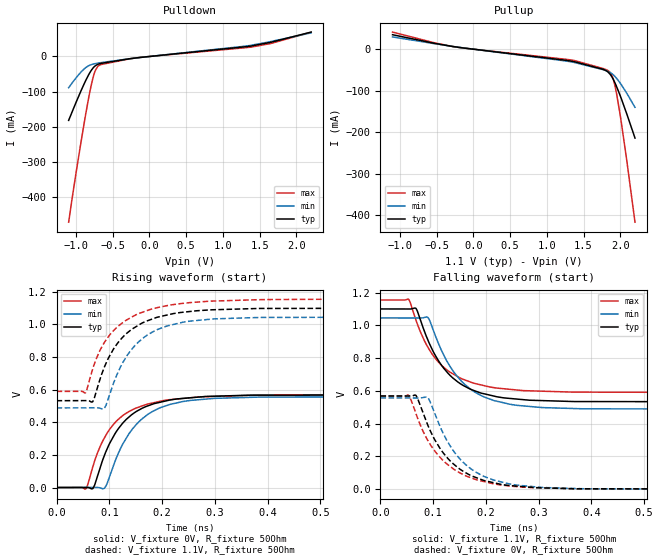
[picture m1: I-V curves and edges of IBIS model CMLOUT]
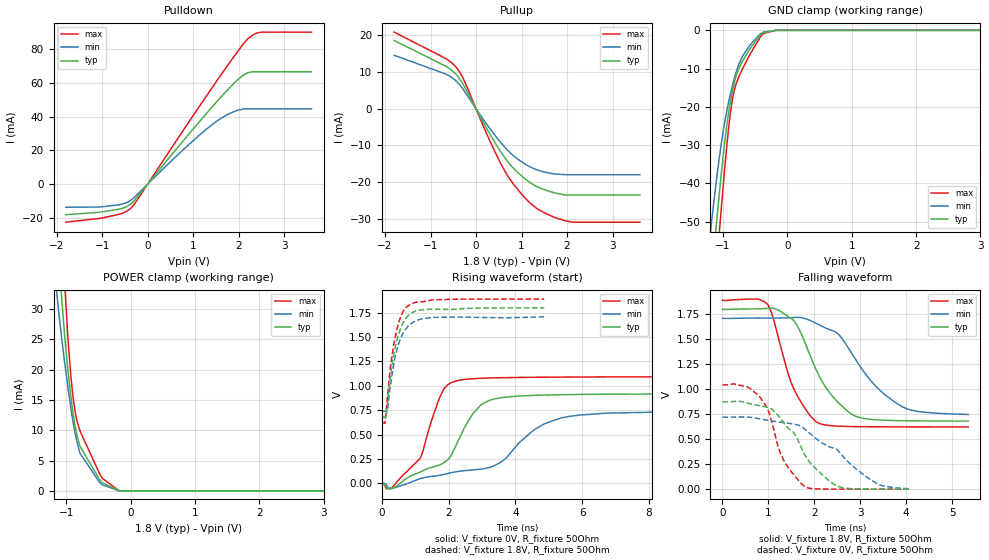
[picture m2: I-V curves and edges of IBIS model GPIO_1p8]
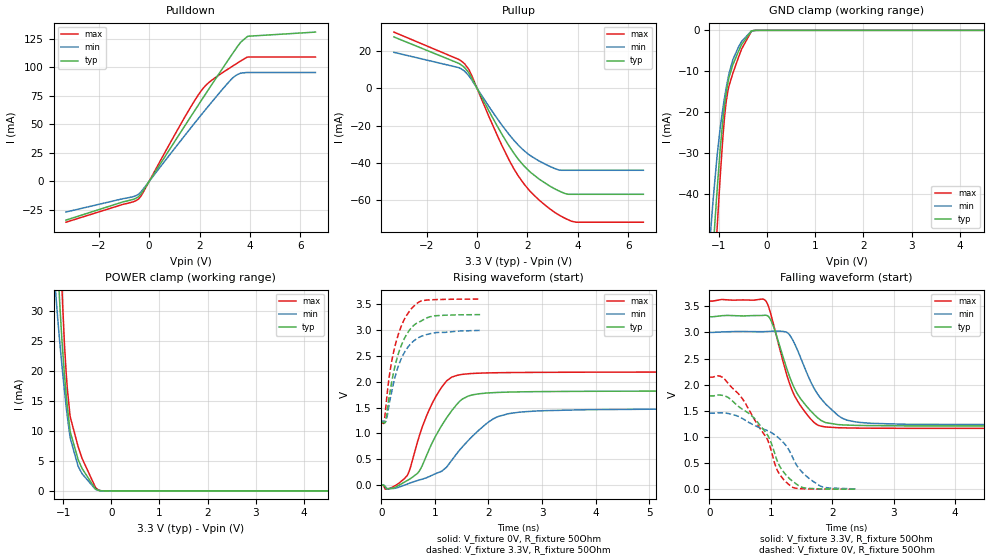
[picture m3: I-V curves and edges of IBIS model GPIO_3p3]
| Texas Instruments Incorporated
| DS90UB9702-Q1 FPD-Link III/IV QuadDeserializer with MIPICSI-2 DPHY out. ports
| Marketing part#   Digital Voltage Range   Package-type   #pins
| DS90UB9702-Q1   1.1V - 3.6V   VQFNP   88
[IBIS Ver]   4.1
[File name]   ds90ub9702-q1.ibs
[File Rev]   1.0
[Date]   05/27/2021
[Source]
| Texas Instruments Incorporated.
| FPD-Link Design and Systems Engineering
| 2900 Semiconductor Driver
| Santa Clara, CA
[Notes]   Revision History:
| Rev 1.0: 05/27/2021
| - Initial version of the model
| - Model generated from simulations in CADENCE
| - Warnings regarding combined Non-monotonicity of various models
|   have been reviewed and considered minor and can be ignored.
| - FPD3_RX, FPD4_RX used in single ended mode
[Disclaimer]
| This model is designed as an aid for customers of Texas Instruments.
| TI and its licensors and suppliers make no warranties, either expressed
| or implied, with respect to this  model, including the warranties of
| merchantability or fitness for a particular purpose. The model is
| provided solely on an "as is" basis. The entire risk as to its quality
| and performance is with the customer.
[Copyright]
(C) Copyright 2021 Texas Instruments Incorporated.All rights reserved.
|   ds90ub9702-q1
[Component]   ds90ub9702-q1
[Manufacturer]   TI
[Package]   |VQFNP 88
|   typ   min   max
R_pkg   0.117   0.089   0.157
L_pkg   2.39nH   1.95nH   3.04nH
C_pkg   0.493pF   0.405pF   0.603pF
[Pin] signal_name  model_name   R_pin  L_pin  C_pin
  1   CML2P   CMLOUT   NA   NA   NA
  2   CML2N   CMLOUT   NA   NA   NA
  3   CML3P   CMLOUT   NA   NA   NA
  4   CML3N   CMLOUT   NA   NA   NA
  5   VDD11_L   power   NA   NA   NA
  6   GPIO0   GPIO   NA   NA   NA
  7   GPIO1   GPIO   NA   NA   NA
  8   GPIO2   GPIO   NA   NA   NA
  9   INTB/GPIO3   GPIO2   NA   NA   NA
 10   LOCK/GPIO4   GPIO   NA   NA   NA
 11   GPIO5   GPIO   NA   NA   NA
 12   GPIO6   GPIO   NA   NA   NA
 13   GPIO7   GPIO   NA   NA   NA
 14   RES   nc   NA   NA   NA
 15   REFCLK   REFCLK   NA   NA   NA
 16  VDDIO   power   NA   NA   NA
 17  CSI2_CLK0N   DPHYTX   NA   NA   NA
 18  CSI2_CLK0P   DPHYTX   NA   NA   NA
 19  CSI2_D0N   DPHYTX   NA   NA   NA
 20  CSI2_D0P   DPHYTX   NA   NA   NA
 21  CSI2_D1N   DPHYTX   NA   NA   NA
 22  CSI2_D1P   DPHYTX   NA   NA   NA
 23  CSI2_CLK1N   DPHYTX   NA   NA   NA
 24  CSI2_CLK1P   DPHYTX   NA   NA   NA
 25  CSI2_D2N   DPHYTX   NA   NA   NA
 26  CSI2_D2P   DPHYTX   NA   NA   NA
 27  CSI2_D3N   DPHYTX   NA   NA   NA
 28  CSI2_D3P   DPHYTX   NA   NA   NA
 29  VDD11_CSI   power   NA   NA   NA
 30  VDD11_CSI   power   NA   NA   NA
 31  CSI0_CLK0N   DPHYTX   NA   NA   NA
 32  CSI0_CLK0P   DPHYTX   NA   NA   NA
 33  CSI0_D0N   DPHYTX   NA   NA   NA
 34  CSI0_D0P   DPHYTX   NA   NA   NA
 35  CSI0_D1N   DPHYTX   NA   NA   NA
 36  CSI0_D1P   DPHYTX   NA   NA   NA
 37  CSI0_CLK1N   DPHYTX   NA   NA   NA
 38  CSI0_CLK1P   DPHYTX   NA   NA   NA
 39  CSI0_D2N   DPHYTX   NA   NA   NA
 40  CSI0_D2P   DPHYTX   NA   NA   NA
 41  CSI0_D3N   DPHYTX   NA   NA   NA
 42  CSI0_D3P   DPHYTX   NA   NA   NA
 43  VDD11_CSI   power   NA   NA   NA
 44  VDD18_P   power   NA   NA   NA
 45  VDD11_P   power   NA   NA   NA
 46  VDD11_CSI   power   NA   NA   NA
 47  CSI1_CLK0N   DPHYTX   NA   NA   NA
 48  CSI1_CLK0P   DPHYTX   NA   NA   NA
 49  CSI1_D0N   DPHYTX   NA   NA   NA
 50  CSI1_D0P   DPHYTX   NA   NA   NA
 51  CSI1_D1N   DPHYTX   NA   NA   NA
 52  CSI1_D1P   DPHYTX   NA   NA   NA
 53  CSI1_CLK1N   DPHYTX   NA   NA   NA
 54  CSI1_CLK1P   DPHYTX   NA   NA   NA
 55  CSI1_D2N   DPHYTX   NA   NA   NA
 56  CSI1_D2P   DPHYTX   NA   NA   NA
 57  CSI1_D3N   DPHYTX   NA   NA   NA
 58  CSI1_D3P   DPHYTX   NA   NA   NA
 59  VDD11_CSI   power   NA   NA   NA
 60  TESTEN   nc   NA   NA   NA
 61  PDB   PDB_18   NA   NA   NA
 62  VDD11_L   power   NA   NA   NA
 63  CML0N   CMLOUT   NA   NA   NA
 64  CML0P   CMLOUT   NA   NA   NA
 65  CML1N   CMLOUT   NA   NA   NA
 66  CML1P   CMLOUT   NA   NA   NA
 67  I2C_SDA   I2C   NA   NA   NA
 68  I2C_SCL   I2C   NA   NA   NA
 69  VDD18_FPD0   power   NA   NA   NA
 70  RIN0+   RIN   NA   NA   NA
 71  RIN0-   RIN   NA   NA   NA
 72  VDD11_FPD   power   NA   NA   NA
 73  RIN1+   RIN   NA   NA   NA
 74  RIN1-   RIN   NA   NA   NA
 75  VDD18_FPD1   power   NA   NA   NA
 76  IDX   nc   NA   NA   NA
 77  LPF   nc   NA   NA   NA
 78  MODE   nc   NA   NA   NA
 79  VDD11_CSI   power   NA   NA   NA
 80  VDD18_FPD2   power   NA   NA   NA
 81  RIN2+   RIN   NA   NA   NA
 82  RIN2-   RIN   NA   NA   NA
 83  VDD11_FPD   power   NA   NA   NA
 84  RIN3+   RIN   NA   NA   NA
 85  RIN3-   RIN   NA   NA   NA
 86  VDD18_FPD3   power   NA   NA   NA
 87  I2C_SCL1/GPIO9  I2C1   NA   NA   NA
 88  I2C_SDA1/GPIO10 I2C1   NA   NA   NA
| RIN model the diff cell line in IBIS needs to be commented
| out to use this model
[Diff pin]  inv_pin  vdiff  tdelay_typ  tdelay_min  tdelay_max
  1   2   0.9   0.0s   0.0s   0.0s
  3   4   0.9   0.0s   0.0s   0.0s
  18  17   0.4   0.0s   0.0s   0.0s
  20  19   0.4   0.0s   0.0s   0.0s
  22  21   0.4   0.0s   0.0s   0.0s
  24  23   0.4   0.0s   0.0s   0.0s
  26  25   0.4   0.0s   0.0s   0.0s
  28  27   0.4   0.0s   0.0s   0.0s
  32  31   0.4   0.0s   0.0s   0.0s
  34  33   0.4   0.0s   0.0s   0.0s
  36  35   0.4   0.0s   0.0s   0.0s
  38  37   0.4   0.0s   0.0s   0.0s
  40  39   0.4   0.0s   0.0s   0.0s
  42  41   0.4   0.0s   0.0s   0.0s
  48  47   0.4   0.0s   0.0s   0.0s
  50  49   0.4   0.0s   0.0s   0.0s
  52  51   0.4   0.0s   0.0s   0.0s
  54  53   0.4   0.0s   0.0s   0.0s
  56  55   0.4   0.0s   0.0s   0.0s
  58  57   0.4   0.0s   0.0s   0.0s
  64  63   0.9   0.0s   0.0s   0.0s
  66  65   0.9   0.0s   0.0s   0.0s
 | 70  71   0.4   0.0s   0.0s   0.0s
 | 73  74   0.4   0.0s   0.0s   0.0s
 | 81  82   0.4   0.0s   0.0s   0.0s
 | 84  85   0.4   0.0s   0.0s   0.0s
|   Model Selectors
[Model Selector] GPIO
GPIO_1p8   1.8V  digital GPIO
GPIO_3p3   3.3V  digital GPIO
[Model Selector] GPIO2
INTB_SHAREIO_18   1.8V digital IO Open Drain Cell
INTB_SHAREIO_33   3.3V digital IO Open Drain Cell
IO_SHAREINTB_18   1.8V digital GPIO for combination with Open Drain Cell
IO_SHAREINTB_33   3.3V digital GPIO for combination with Open Drain Cell
[Model Selector] REFCLK
REFCLK_18   REFCLK 1.8v
REFCLK_33   REFCLK 3.3v
[Model Selector] I2C
I2C_FAST_33   I2C FAST 3.3v
I2C_FAST_18   I2C FAST 1.8v
I2C_FASTPLUS_33   I2C FASTPLUS 3.3v
I2C_FASTPLUS_18   I2C FASTPLUS 1.8v
[Model Selector] I2C1
I2C_FAST_33   I2C FAST 3.3v
I2C_FAST_18   I2C FAST 1.8v
I2C_FASTPLUS_33   I2C FASTPLUS 3.3v
I2C_FASTPLUS_18   I2C FASTPLUS 1.8v
GPIO2_1p8   1.8V digital GPIO for combination with Open Drain Cell
GPIO2_3p3   1.8V digital GPIO for combination with Open Drain Cell
[Model Selector] DPHYTX
DPHY_HS   DPHY Tx HS
DPHY_LP   DPHY Tx LP
[Model Selector] RIN
FPD3_RX   FPD-Link 3 Receiver-Transmitter
FPD4_RX   FPD-Link 4 Receiver-Transmitter
| Models and submodels in the file (20): CMLOUT (Output), GPIO_1p8 (I/O), GPIO_3p3 (I/O), GPIO2_1p8 (I/O), GPIO2_3p3 (I/O), REFCLK_18 (Input), REFCLK_33 (Input), I2C_FAST_18 (I/O_open_drain), I2C_FAST_33 (I/O_open_drain), I2C_FASTPLUS_18 (I/O_open_drain), I2C_FASTPLUS_33 (I/O_open_drain), PDB_18 (Input), DPHY_HS (Output), DPHY_LP (Output), INTB_SHAREIO_18 (I/O_open_drain), INTB_SHAREIO_33 (I/O_open_drain), IO_SHAREINTB_18 (I/O), IO_SHAREINTB_33 (I/O), FPD3_RX (I/O), FPD4_RX (I/O)
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|   CMLOUT Model
[Model]   CMLOUT
Model_type   Output
Polarity   Non-Inverting
Vmeas = 0.55
Vref = 0.55
Cref = 0pF
Rref = 50
|   typ   min   max
C_comp   1.329pF   1.392pF   1.158pF
[Voltage Range]   1.1   1.045   1.155
[Temperature Range]   27   105   -40
[Pullup Reference]   1.1   1.045   1.155
[Pulldown Reference]   -0   -0   0
[Power Clamp Reference]   1.1   1.045   1.155
[GND Clamp Reference]   0   0   0
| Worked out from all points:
|   slope of the pulldown table from 0 to 0.165 V, typ, clamps not added: 46.5 ohm
|   slope of the pullup table from 0 to 0.165 V, typ, clamps not added: 46.5 ohm
|   falling waveform, V_fixture 1.1V, R_fixture 50Ohm: 20-80 % time 69.8ps typ, 71.3ps min, 72.1ps max; typ from 1.1 V to 0.532 V
|   rising waveform, V_fixture 0V, R_fixture 50Ohm: 20-80 % time 64.2ps typ, 66.4ps min, 64.3ps max; typ from 0.001 V to 0.569 V
|   rising waveform, V_fixture 1.1V, R_fixture 50Ohm: 20-80 % time 70.5ps typ, 67.9ps min, 74.8ps max; typ from 0.532 V to 1.1 V
|   falling waveform, V_fixture 0V, R_fixture 50Ohm: 20-80 % time 72.5ps typ, 72.3ps min, 75.1ps max; typ from 0.569 V to 0.001 V
[Pulldown]
|   Voltage   I(typ)   I(min)   I(max)
-1.1V     -182.3mA   -89mA      -472.7mA
-1.05V    -156.9mA   -74.89mA   -401.7mA
-931.7mV  -97.86mA   -44.34mA   -243.8mA
-829.4mV  -52.8mA    -26.56mA   -120.1mA
-793.1mV  -39.97mA   -23.28mA   -82.45mA
-756.8mV  -30.23mA   -21.16mA   -52.03mA
-737mV    -26.5mA    -20.27mA   -40.1mA
-694.1mV  -21.7mA    -18.66mA   -26.62mA
-136.4mV  -3.021mA   -3.195mA   -2.891mA
1.382V    29.73mA    31.87mA    26.64mA
1.662V    41.07mA    43.15mA    37.62mA
2.2V      69.57mA    67.39mA    69.39mA
[Pullup]
|   Voltage   I(typ)   I(min)   I(max)
-1.1V     34.88mA    29.53mA    41.23mA
-235.4mV  5.289mA    5.509mA    5.07mA
1.335V    -29.01mA   -30.79mA   -26.25mA
1.764V    -48.67mA   -49.31mA   -46.6mA
1.83V     -54.84mA   -53.46mA   -51.41mA
1.86V     -60.26mA   -56.13mA   -55.69mA
1.893V    -69.21mA   -60.2mA    -66.46mA
1.923V    -79.58mA   -65.05mA   -84.76mA
1.949V    -90.16mA   -70.26mA   -107.3mA
2.012V    -118.5mA   -85.19mA   -174.6mA
2.091V    -157.7mA   -107.2mA   -272.5mA
2.2V      -214.5mA   -140.3mA   -417.4mA
[Ramp]
R_load = 50
|   typ   min   max
dV/dt_r   0.341018/6.43645e-11   0.333768/6.66287e-11   0.340926/6.43299e-11
dV/dt_f   0.340493/6.98585e-11   0.334059/7.13859e-11   0.339127/7.12696e-11
[Falling Waveform]
V_fixture = 1.1V
V_fixture_min = 1.045V
V_fixture_max = 1.155V
R_fixture = 50Ohm
C_fixture = 0F
|   Time   V(typ)   V(min)   V(max)
0s        1.1V       1.045V     1.154V
53.68ps   1.099V     1.045V     1.158V
67.79ps   1.102V     1.045V     1.029V
89.79ps   912.7mV    1.049V     868.1mV
113.7ps   766.3mV    862.1mV    763.2mV
140.1ps   671.9mV    711.6mV    699.3mV
171ps     610.4mV    610.6mV    654mV
207ps     574.6mV    550.8mV    624.2mV
384.8ps   534.9mV    490.7mV    592.2mV
1ns       532.3mV    488.1mV    589.2mV
[Rising Waveform]
V_fixture = 0V
V_fixture_min = 0V
V_fixture_max = 0V
R_fixture = 50Ohm
C_fixture = 0F
|   Time   V(typ)   V(min)   V(max)
0s        540.9uV    677.7uV    610.6uV
55.55ps   1.062mV    1.133mV    -7.529mV
69.19ps   -4.06mV    1.245mV    131.9mV
90.63ps   196.2mV    -4.053mV   304mV
113.7ps   345.1mV    184.3mV    407.7mV
140.1ps   440mV      342.7mV    470.4mV
171ps     498.1mV    443.7mV    510.1mV
200.6ps   525.9mV    493.7mV    531.7mV
384.8ps   566.1mV    554.4mV    565.9mV
1ns       568.9mV    557mV      568.8mV
[Rising Waveform]
V_fixture = 1.1V
V_fixture_min = 1.045V
V_fixture_max = 1.155V
R_fixture = 50Ohm
C_fixture = 0F
|   Time   V(typ)   V(min)   V(max)
0s        532.2mV    488.1mV    589.2mV
54.91ps   532.7mV    488.5mV    580.6mV
68.52ps   525.9mV    488.6mV    726mV
89.79ps   730.4mV    482.7mV    883.6mV
120ps     901.1mV    731mV      996.6mV
140.1ps   963.1mV    837.3mV    1.039V
175.2ps   1.025V     940.7mV    1.088V
221.3ps   1.065V     998.7mV    1.121V
384.8ps   1.097V     1.042V     1.151V
1ns       1.1V       1.045V     1.154V
[Falling Waveform]
|Gnd
V_fixture = 0V
V_fixture_min = 0V
V_fixture_max = 0V
R_fixture = 50Ohm
C_fixture = 0F
|   Time   V(typ)   V(min)   V(max)
0s        568.9mV    557mV      568.8mV
53.37ps   568.6mV    556.8mV    573.8mV
67.98ps   569.9mV    556.7mV    457mV
89.29ps   396mV      561mV      301.3mV
113.7ps   246mV      378.3mV    193mV
143.7ps   140.6mV    211.8mV    113.4mV
175.2ps   78.68mV    116.6mV    65.93mV
213.7ps   40.69mV    57.28mV    33.78mV
384.8ps   2.882mV    3.195mV    2.937mV
1ns       541uV      676.8uV    609.5uV
|   GPIO_1p8 Model
[Model]   GPIO_1p8
Model_type   I/O
Polarity   Non-Inverting
Enable   Active-Low
Vinl = 0.63
Vinh = 1.17
Vmeas = 0.9
Vref = 0
Cref = 2pF
Rref = 80
|   typ   min   max
|   (nom PVT)   (fast PVT)   (slow PVT)
C_comp   3.718e-13   3.701e-13   4.153e-13
| Where nom  PVT is Nominal Process, 1.8V, 27C
|   Fast PVT is Strong Process,  1.89V, -40C
|   Slow PVT is Weak Process,   1.71V, 125C
[Voltage Range]   1.8   1.71   1.89
|Junction Temperature
[Temperature Range]   27   125   -40
[Pullup Reference]   1.8   1.71   1.89
[Pulldown Reference]   0   0   0
[Power Clamp Reference]   1.8   1.71   1.89
[GND Clamp Reference]   0   0   0
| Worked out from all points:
|   slope of the pulldown table from 0 to 0.27 V, typ, clamps not added: 30.2 ohm
|   slope of the pullup table from 0 to 0.27 V, typ, clamps not added: 43.9 ohm
|   GND clamp passes 1 mA (typ) near -0.40 V on its own axis
|   falling waveform, V_fixture 1.8V, R_fixture 50Ohm: 20-80 % time 748ps typ, 967ps min, 555ps max; typ from 1.8 V to 0.682 V
|   rising waveform, V_fixture 0V, R_fixture 50Ohm: 20-80 % time 1.1ns typ, 1.78ns min, 675ps max; typ from 0 V to 0.874 V
|   rising waveform, V_fixture 1.8V, R_fixture 50Ohm: 20-80 % time 358ps typ, 369ps min, 331ps max; typ from 0.681 V to 1.8 V
|   falling waveform, V_fixture 0V, R_fixture 50Ohm: 20-80 % time 824ps typ, 1.21ns min, 503ps max; typ from 0.875 V to 0 V
[Pulldown]
|   Voltage   I(typ)   I(min)   I(max)
-1.8V     -18.1mA    -13.7mA    -22.52mA
-1.118V   -16.75mA   -13.57mA   -20.48mA
-616.7mV  -14.76mA   -12.18mA   -17.81mA
-370.8mV  -11.74mA   -9.537mA   -14.3mA
682.9mV   22.51mA    17.91mA    27.88mA
1.375V    44.46mA    34.38mA    55.51mA
1.806V    57.22mA    41.87mA    72.16mA
2.108V    64.69mA    44.51mA    83.23mA
2.222V    66.11mA    44.62mA    86.57mA
2.351V    66.54mA    44.62mA    88.92mA
2.507V    66.54mA    44.62mA    90.02mA
3.6V      66.54mA    44.62mA    90.04mA
[GND Clamp]
|   Voltage   I(typ)   I(min)   I(max)
-1.8V     -186.8mA   -154.6mA   -219.7mA
-1.184V   -65.39mA   -50.91mA   -80.03mA
-1.142V   -57.47mA   -44.58mA   -70.68mA
-1.093V   -48.73mA   -37.8mA    -60.24mA
-1.032V   -38.28mA   -30.14mA   -47.51mA
-918mV    -21.99mA   -19.11mA   -26.27mA
-867.6mV  -16.94mA   -15.37mA   -19.43mA
-826.6mV  -13.75mA   -12.69mA   -15.72mA
-692.5mV  -7.885mA   -6.615mA   -9.905mA
-371.2mV  -556.1uA   -459.4uA   -815.6uA
-180mV    -2.088uA   -5.52uA    -1.102uA
3.6V      0A         0A         0A
[Pullup]
|   Voltage   I(typ)   I(min)   I(max)
-1.8V     18.57mA    14.55mA    20.87mA
-687.6mV  11.7mA     9.532mA    13.79mA
-427.9mV  9.197mA    7.405mA    11.15mA
-295.6mV  6.918mA    5.493mA    8.587mA
252mV     -5.809mA   -4.572mA   -7.364mA
467.5mV   -10.33mA   -8.117mA   -13.11mA
628.7mV   -13.33mA   -10.48mA   -16.92mA
951.8mV   -17.82mA   -14.11mA   -22.6mA
1.319V    -21.16mA   -16.61mA   -27.08mA
1.761V    -23.08mA   -17.88mA   -29.82mA
2.117V    -23.57mA   -18.03mA   -30.96mA
3.6V      -23.57mA   -18.03mA   -30.98mA
[POWER Clamp]
|   Voltage   I(typ)   I(min)   I(max)
-1.8V     198.5mA    148.8mA    248.5mA
-1.154V   45.96mA    33.07mA    64.85mA
-1.133V   41.99mA    30.87mA    59.48mA
-1.076V   32.34mA    25.46mA    45.52mA
-1.018V   24.38mA    20.39mA    32.58mA
-930.6mV  15.62mA    13.69mA    19.01mA
-889mV    12.28mA    10.92mA    14.86mA
-849.6mV  9.776mA    8.708mA    12.16mA
-783.2mV  7.264mA    6.117mA    9.767mA
-443mV    1.357mA    1.021mA    2.096mA
-180mV    9.68uA     16.22uA    11.61uA
3.6V      0A         0A         0A
[Ramp]
R_load = 50
|   typ   min   max
dV/dt_r   0.524217/1.09833e-09   0.43397/1.76732e-09   0.626665/6.67214e-10
dV/dt_f   0.671532/7.48876e-10   0.581643/9.8061e-10   0.760362/5.53965e-10
[Falling Waveform]
V_fixture = 1.8V
V_fixture_min = 1.71V
V_fixture_max = 1.89V
R_fixture = 50Ohm
|   Time   V(typ)   V(min)   V(max)
0s        1.8V       1.71V      1.89V
766.7ps   1.805V     1.714V     1.904V
989ps     1.811V     1.713V     1.846V
1.533ns   1.697V     1.718V     1.025V
2.044ns   1.193V     1.66V      673.8mV
2.515ns   870.7mV    1.556V     631.5mV
2.96ns    720.5mV    1.255V     626.2mV
3.429ns   692.8mV    990.2mV    624.5mV
3.917ns   685.9mV    824.1mV    623.6mV
5.349ns   681.6mV    748.2mV    622.9mV
[Rising Waveform]
V_fixture = 0V
V_fixture_min = 0V
V_fixture_max = 0V
R_fixture = 50Ohm
|   Time   V(typ)   V(min)   V(max)
0s        1.128uV    5.641uV    494.5nV
262.6ps   -52.87mV   -47.73mV   -51.45mV
1.143ns   115.5mV    49.48mV    254.9mV
1.673ns   182.1mV    80.13mV    829.4mV
1.983ns   247.2mV    103.2mV    1.014V
2.976ns   808.6mV    146.4mV    1.078V
4.521ns   902.3mV    539.1mV    1.088V
6.688ns   914.5mV    719.5mV    1.092V
13.35ns   920.1mV    749mV      1.092V
300ns     873.7mV    723.3mV    1.044V
[Rising Waveform]
V_fixture = 1.8V
V_fixture_min = 1.71V
V_fixture_max = 1.89V
R_fixture = 50Ohm
|   Time   V(typ)   V(min)   V(max)
0s        680.7mV    740.6mV    622.7mV
100.4ps   673.9mV    740.5mV    631.3mV
133.3ps   701.5mV    734.3mV    750.6mV
158.8ps   785.6mV    747.9mV    860.5mV
282.6ps   1.165V     1.063V     1.257V
421ps     1.427V     1.332V     1.535V
586.7ps   1.609V     1.506V     1.727V
766.7ps   1.712V     1.603V     1.815V
1.469ns   1.786V     1.7V       1.879V
4.861ns   1.799V     1.708V     1.89V
[Falling Waveform]
V_fixture = 0V
V_fixture_min = 0V
V_fixture_max = 0V
R_fixture = 50Ohm
|   Time   V(typ)   V(min)   V(max)
0s        874.5mV    720.8mV    1.045V
532.1ps   863.9mV    722.2mV    1.025V
806ps     836.4mV    704.8mV    927.6mV
1.012ns   814.7mV    687.4mV    770.3mV
1.322ns   671.5mV    667.4mV    299.7mV
1.574ns   551.2mV    649.8mV    132.5mV
1.79ns    347.4mV    602.3mV    25.61mV
2.501ns   29.95mV    394.8mV    605.9uV
3.341ns   717uV      61.55mV    228.3uV
4.053ns   251.3uV    4.228mV    121.4uV
|   GPIO_3p3 Model
[Model]   GPIO_3p3
Model_type   I/O
Polarity   Non-Inverting
Enable   Active-Low
Vinl = 0.8
Vinh = 2
Vmeas = 1.65
Vref = 0
Cref = 2pF
Rref = 100
|   typ   min   max
|   (nom PVT)   (fast PVT)   (slow PVT)
C_comp   3.371e-13   3.361e-13   3.845e-13
| Where nom  PVT is Nominal Process, 3.3V, 27C
|   Fast PVT is Strong Process,  3.6V, -40C
|   Slow PVT is Weak Process,   3V, 125C
[Voltage Range]   3.3   3   3.6
|Junction Temperature
[Temperature Range]   27   125   -40
[Pullup Reference]   3.3   3   3.6
[Pulldown Reference]   0   0   0
[Power Clamp Reference]   3.3   3   3.6
[GND Clamp Reference]   0   0   0
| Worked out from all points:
|   slope of the pulldown table from 0 to 0.495 V, typ, clamps not added: 29 ohm
|   slope of the pullup table from 0 to 0.495 V, typ, clamps not added: 38.9 ohm
|   GND clamp passes 1 mA (typ) near -0.38 V on its own axis
|   falling waveform, V_fixture 3.3V, R_fixture 50Ohm: 20-80 % time 444ps typ, 490ps min, 388ps max; typ from 3.3 V to 1.21 V
|   rising waveform, V_fixture 0V, R_fixture 50Ohm: 20-80 % time 558ps typ, 789ps min, 456ps max; typ from 0 V to 1.8 V
|   rising waveform, V_fixture 3.3V, R_fixture 50Ohm: 20-80 % time 319ps typ, 328ps min, 291ps max; typ from 1.21 V to 3.3 V
|   falling waveform, V_fixture 0V, R_fixture 50Ohm: 20-80 % time 526ps typ, 688ps min, 536ps max; typ from 1.79 V to 0.001 V
[Pulldown]
|   Voltage   I(typ)   I(min)   I(max)
-3.3V     -33.8mA    -26.73mA   -35.63mA
-621mV    -15.55mA   -13.2mA    -17.7mA
-416.4mV  -13.15mA   -11.02mA   -15.19mA
-243.6mV  -8.298mA   -6.901mA   -9.764mA
1.479V    50.9mA     42.06mA    58.86mA
2.057V    70.47mA    58.02mA    79.16mA
2.436V    83.19mA    68.27mA    87.87mA
3.303V    111.7mA    90.39mA    100.9mA
3.623V    121.6mA    94.78mA    105.4mA
3.871V    126.5mA    95.44mA    108.7mA
3.925V    127.2mA    95.44mA    109mA
6.6V      130.8mA    95.44mA    109mA
[GND Clamp]
|   Voltage   I(typ)   I(min)   I(max)
-3.3V     -491.8mA   -423.9mA   -559.8mA
-1.239V   -75.42mA   -59.14mA   -91.74mA
-1.131V   -55.26mA   -42.87mA   -68mA
-1.118V   -52.97mA   -41.09mA   -65.28mA
-1.035V   -38.5mA    -30.32mA   -47.74mA
-916.8mV  -21.68mA   -18.91mA   -25.82mA
-858mV    -16mA      -14.63mA   -18.24mA
-808.8mV  -12.51mA   -11.55mA   -14.49mA
-711mV    -8.408mA   -7.158mA   -10.49mA
-597mV    -5.192mA   -4.144mA   -6.684mA
-330mV    -214.7uA   -206.3uA   -301.9uA
6.6V      0A         0A         0A
[Pullup]
|   Voltage   I(typ)   I(min)   I(max)
-3.3V     27.38mA    19.16mA    29.98mA
-726mV    13.26mA    10.98mA    15.37mA
-495mV    11.02mA    9.082mA    13.04mA
-214.8mV  5.559mA    4.494mA    6.876mA
858mV     -21.64mA   -17.37mA   -26.91mA
1.461V    -34.78mA   -27.84mA   -43.1mA
2.13V     -45.07mA   -36.2mA    -55.48mA
2.883V    -52.3mA    -41.79mA   -64.48mA
3.245V    -54.91mA   -43.73mA   -67.77mA
3.513V    -56.41mA   -43.89mA   -69.71mA
3.92V     -56.73mA   -43.89mA   -71.65mA
6.6V      -56.73mA   -43.89mA   -71.65mA
[POWER Clamp]
|   Voltage   I(typ)   I(min)   I(max)
-3.3V     582.6mA    466.3mA    697.7mA
-1.155V   45.95mA    33.1mA     64.9mA
-1.089V   34.1mA     26.51mA    48.26mA
-1.072V   31.39mA    24.93mA    44.12mA
-1.023V   24.87mA    20.75mA    33.46mA
-1.014V   23.81mA    20.01mA    31.67mA
-975mV    19.64mA    16.9mA     24.86mA
-937.2mV  16.08mA    14.08mA    19.71mA
-852mV    9.838mA    8.778mA    12.31mA
-660mV    4.699mA    3.657mA    6.688mA
-306.9mV  228.3uA    200.3uA    413.1uA
6.6V      0A         0A         0A
[Ramp]
R_load = 50
|   typ   min   max
dV/dt_r   1.07754/5.57178e-10   0.880333/7.80725e-10  1.29209/4.54918e-10
dV/dt_f   1.25195/4.43147e-10   1.0571/4.86178e-10   1.43998/3.87318e-10
[Falling Waveform]
V_fixture = 3.3V
V_fixture_min = 3V
V_fixture_max = 3.6V
R_fixture = 50Ohm
|   Time   V(typ)   V(min)   V(max)
0s        3.3V       3V         3.6V
911.5ps   3.328V     3.016V     3.612V
1.037ns   3.133V     3.023V     3.186V
1.252ns   2.34V      3.005V     2.222V
1.413ns   1.867V     2.719V     1.732V
1.75ns    1.38V      1.843V     1.239V
2.086ns   1.237V     1.419V     1.177V
2.38ns    1.222V     1.287V     1.17V
3.221ns   1.212V     1.242V     1.165V
39.35ns   1.213V     1.237V     1.199V
[Rising Waveform]
V_fixture = 0V
V_fixture_min = 0V
V_fixture_max = 0V
R_fixture = 50Ohm
|   Time   V(typ)   V(min)   V(max)
0s        975nV      4.518uV    2.409uV
133.5ps   -66.43mV   -75.67mV   -75.59mV
483.2ps   88.32mV    19.26mV    187.9mV
841.1ps   567.4mV    141.6mV    1.334V
1.221ns   1.304V     351.6mV    2.018V
1.515ns   1.666V     742mV      2.141V
2.032ns   1.785V     1.241V     2.171V
2.95ns    1.808V     1.436V     2.18V
7.921ns   1.821V     1.476V     2.187V
100ns     1.796V     1.467V     2.153V
[Rising Waveform]
V_fixture = 3.3V
V_fixture_min = 3V
V_fixture_max = 3.6V
R_fixture = 50Ohm
|   Time   V(typ)   V(min)   V(max)
0s        1.213V     1.238V     1.2V
46.2ps    1.203V     1.237V     1.195V
80.35ps   1.244V     1.228V     1.501V
154.8ps   1.763V     1.627V     2.163V
265.9ps   2.356V     2.136V     2.739V
379.1ps   2.721V     2.464V     3.096V
548.9ps   3.031V     2.735V     3.399V
719.8ps   3.162V     2.866V     3.551V
990ps     3.273V     2.945V     3.586V
1.853ns   3.297V     2.993V     3.598V
[Falling Waveform]
V_fixture = 0V
V_fixture_min = 0V
V_fixture_max = 0V
R_fixture = 50Ohm
|   Time   V(typ)   V(min)   V(max)
0s        1.786V     1.454V     2.144V
243.2ps   1.787V     1.459V     2.111V
535.8ps   1.531V     1.355V     1.735V
721.6ps   1.37V      1.228V     1.358V
955.4ps   1.019V     1.115V     923.1mV
1.116ns   510.5mV    993.2mV    341mV
1.315ns   191.7mV    708.1mV    69.07mV
1.504ns   37.06mV    333.8mV    8.848mV
1.796ns   6.572mV    66.51mV    2.073mV
2.38ns    1.093mV    5.381mV    722.9uV
